(* Logix 5000 DataType export PacketPower_EnvironmentalMonitor; software revision 33.00 *)

TYPE PacketPower_EnvironmentalMonitor :
STRUCT
   Status : DINT; {access Read Only}   // Power node #1: status mask [1 indicates presence: B0:node, B1-12:temperature probes 1-12
   DataAge : DINT; {access Read Only}   // Data age [s]
   Temperature : REAL; {access Read Only}   // Cel
   RelativeHumidity : REAL; {access Read Only}   // Perc
   ProbeTemperature : REAL[12];   // Cel
END_STRUCT
END_TYPE
